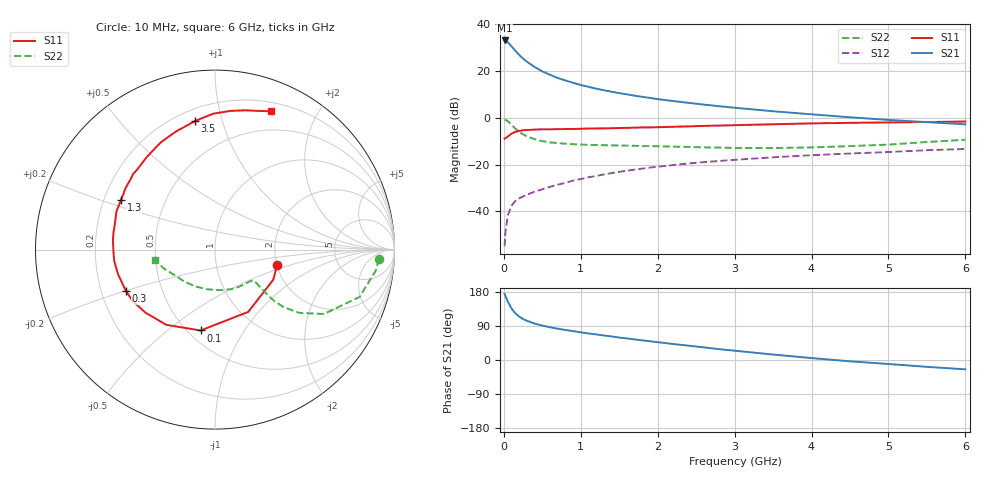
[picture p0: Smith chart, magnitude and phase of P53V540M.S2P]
! SIEMENS Small Signal Semiconductors
! BFP183
! Si NPN RF Bipolar Junction Transistor in SOT143
! VCE = 3.5 V  IC = 40 mA
! Common Emitter S-Parameters:  March  1996
# GHz  S  MA  R  50
!  f  S11  S21  S12  S22
! GHz  MAG  ANG  MAG  ANG  MAG  ANG  MAG  ANG
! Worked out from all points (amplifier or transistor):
!   36 points, 10 MHz to 6 GHz, reference 50 ohm
!   highest |S21| = 33.0 dB at 10 MHz (marker M1)
!   |S21| within 3 dB of that: start of sweep to 112.6 MHz
!   unconditionally stable (mu >= 1): 480 MHz to 5.871 GHz
!   at 250 MHz: K = 0.70, MSG = 29.5 dB, |S12| = -33.6 dB
!   at 1.4 GHz: K = 1.25, MAG = 14.4 dB, |S12| = -23.7 dB
!   at 6 GHz: K = 0.98, MSG = 5.3 dB, |S12| = -13.4 dB
!   S11 on the Smith chart (normalised r, x): 10 MHz: 2.01, -0.38; 100 MHz: 0.58, -0.66; 300 MHz: 0.31, -0.20; 1.3 GHz: 0.27, +0.23; 3.5 GHz: 0.27, +0.82; 6 GHz: 0.29, +1.44
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0.01  0.3563 -13.5  44.84 174.5  0.0018 81.7  0.915 -3.3
0.02  0.3656 -27.3  44.68 169.6  0.0035 82.2  0.9035 -7.4
0.05  0.3933 -61.9  41.46 154.7  0.008 72.6  0.8477 -18.1
0.1  0.4578 -100.1  33.54 135.9  0.0132 57.3  0.7051 -30.6
0.15  0.4992 -122.9  26.95 123.2  0.0167 53.1  0.5871 -36.9
0.2  0.5232 -137.9  22.02 114.4  0.0189 52.2  0.5006 -39.9
0.25  0.5407 -148.0  18.38 108.1  0.0208 51.0  0.4417 -40.9
0.3  0.5473 -155.1  15.76 103.5  0.0227 52.0  0.3992 -40.9
0.4  0.5575 -165.8  12.15 96.1  0.0263 53.7  0.3473 -40.2
0.5  0.5655 -173.8  9.796 90.9  0.0296 55.5  0.3167 -39.5
0.6  0.5662 -179.5  8.293 86.5  0.0334 57.0  0.2981 -39.0
0.7  0.5712 174.7  7.086 82.6  0.0371 58.3  0.2863 -38.8
0.8  0.5735 170.4  6.264 79.2  0.0406 58.9  0.2788 -39.2
1.1  0.5887 158.9  4.58 70.0  0.0534 59.5  0.2636 -41.8
1.3  0.5926 152.2  3.865 64.7  0.0614 58.7  0.2591 -44.7
1.7  0.6128 139.8  2.956 54.4  0.0779 56.5  0.2514 -51.9
2.2  0.6402 126.6  2.272 42.3  0.0974 52.5  0.2409 -62.9
2.8  0.6796 112.5  1.764 28.6  0.1191 46.7  0.2304 -79.2
3.5  0.7249 98.8  1.376 14.4  0.1426 40.1  0.2254 -101.0
4.5  0.7774 83.7  1.023 -3.5  0.1719 30.6  0.2471 -134.2
5.5  0.8085 72.9  0.806 -18.1  0.2024 22.1  0.303 -159.4
6  0.8308 68.1  0.723 -24.6  0.215 17.3  0.3386 -170.2
